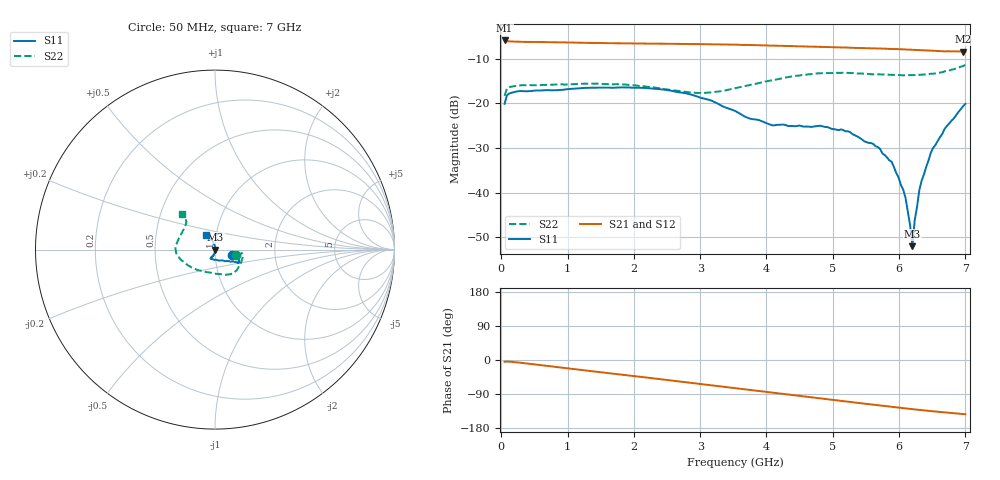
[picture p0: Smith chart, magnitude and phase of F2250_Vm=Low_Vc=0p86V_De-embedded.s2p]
! Integrated Device Technology
! Corporate Headquarters
! 6024 Silver Creek Valley Road
! San Jose, CA 95138  USA
! Phone:  1-408-284-8200
! Toll Free:  1-800-223-1366
! Webpage:  http://www.idt.com/
! Timing and RF Division
! 515 Groton Road, Suite 102
! Westford, MA 01886-6024
! Device:  F2250
! Description: Voltage Variable RF Attenuator
! Frequency:  50.0 -  6000.00 MHz
! Package:  3x3 mm Thin QFN Plastic Package: 16 pin
! Ports:  2 RF, 3 DC
!  Pin  1  = GND
!  Pin  2  = NC
!  Pin  3  = RF1  = Port 1
!  Pin  4  = NC
!  Pin  5  = GND
!  Pin  6  = GND
!  Pin  7  = GND
!  Pin  8  = GND
!  Pin  9  = NC
!  Pin 10  = RF2  = Port 2
!  Pin 11  = NC
!  Pin 12  = GND
!  Pin 13  = GND
!  Pin 14  = VCNTRL
!  Pin 15  = VDD
!  Pin 16  = VMODE
! Vcntrl:  0.860 Volts
! Vmode:  +0.000 Volts
! Vdd:  +3.30  Volts
! Current:  1.173 mA
! Data:  The device was measured on a the F2250 evaluation board which has
!  individual transmission lines to the RF pins.  Data was collected
!  using a calibrated network analyzer.  The evaluation board was
!  de-embedded using a TRL calibration technique.
!  The reference plane is the edge of the package pin.
! Misc:  SN 10
!  Action Tracker AT0258
! Date Measured:  2014-11-26
! Date:  2015-10-15  MJV
! Note:
!  Integrated Device Technology supplies this data as a sample of measured
!  data at the package pin for this product.  Your particular data for this
!  product may vary.
!  Data was taken at 25 degrees C.
!  Integrated Device Technology reserves the right to change this data at anytime.
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# GHz S dB R 50
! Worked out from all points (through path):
!   201 points, 50 MHz to 7 GHz, reference 50 ohm
!   highest |S21| = -5.89 dB at 50 MHz (marker M1); lowest = -8.4 dB at 6.965 GHz (marker M2)
!   group delay of S21, straight-line fit = 57.3 ps
!   lowest |S11| = -52.0 dB at 6.201 GHz (marker M3), VSWR 1.01, Z = 50.3 + j0.0375 ohm
!   |S11| at or under -10 dB: start of sweep to end of sweep
!   |S22| runs from -18.3 to -11.4 dB; largest |S21 - S12| = 0.0013
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0.05  -20.08 -18.9  -5.89 -4.8  -5.89 -4.8  -18.30 -15.0
0.08475  -18.18 -9.8  -6.06 -4.2  -6.04 -4.2  -16.64 -8.8
0.22375  -17.35 -7.7  -6.17 -6.0  -6.15 -6.0  -16.07 -10.3
1.2315  -16.55 -25.3  -6.41 -26.8  -6.41 -26.8  -15.57 -42.6
2.37825  -16.78 -29.9  -6.62 -50.2  -6.63 -50.2  -16.58 -70.0
3.0385  -18.85 -35.7  -6.71 -64.1  -6.72 -64.1  -17.67 -100.9
3.525  -21.67 -50.4  -6.84 -74.5  -6.83 -74.5  -16.59 -129.5
4.081  -24.88 -83.5  -7.05 -86.3  -7.05 -86.3  -14.83 -154.9
4.7065  -25.18 -113.9  -7.29 -99.4  -7.29 -99.4  -13.40 -172.9
5.2625  -26.45 -113.6  -7.53 -110.8  -7.54 -110.8  -13.17 174.5
5.6795  -29.76 -103.8  -7.69 -119.3  -7.69 -119.3  -13.49 164.0
5.85325  -32.76 -96.9  -7.79 -122.7  -7.78 -122.8  -13.58 159.5
5.99225  -36.57 -94.2  -7.85 -125.6  -7.84 -125.6  -13.65 155.4
6.0965  -41.08 -81.1  -7.92 -127.6  -7.93 -127.6  -13.68 152.0
6.166  -47.28 -48.0  -7.96 -129.0  -7.96 -129.0  -13.67 149.6
6.20075  -51.97 8.5  -7.99 -129.7  -7.99 -129.7  -13.64 148.5
6.2355  -46.15 51.5  -8.01 -130.3  -8.02 -130.4  -13.66 147.2
6.305  -39.42 87.8  -8.05 -131.7  -8.06 -131.7  -13.58 145.0
6.47875  -31.03 98.3  -8.17 -134.9  -8.18 -134.9  -13.34 139.9
6.68725  -25.68 106.6  -8.33 -138.2  -8.32 -138.3  -12.81 134.7
6.96525  -20.64 121.0  -8.40 -142.6  -8.39 -142.7  -11.61 133.6
7  -20.09 122.0  -8.40 -143.1  -8.39 -143.2  -11.42 133.2
